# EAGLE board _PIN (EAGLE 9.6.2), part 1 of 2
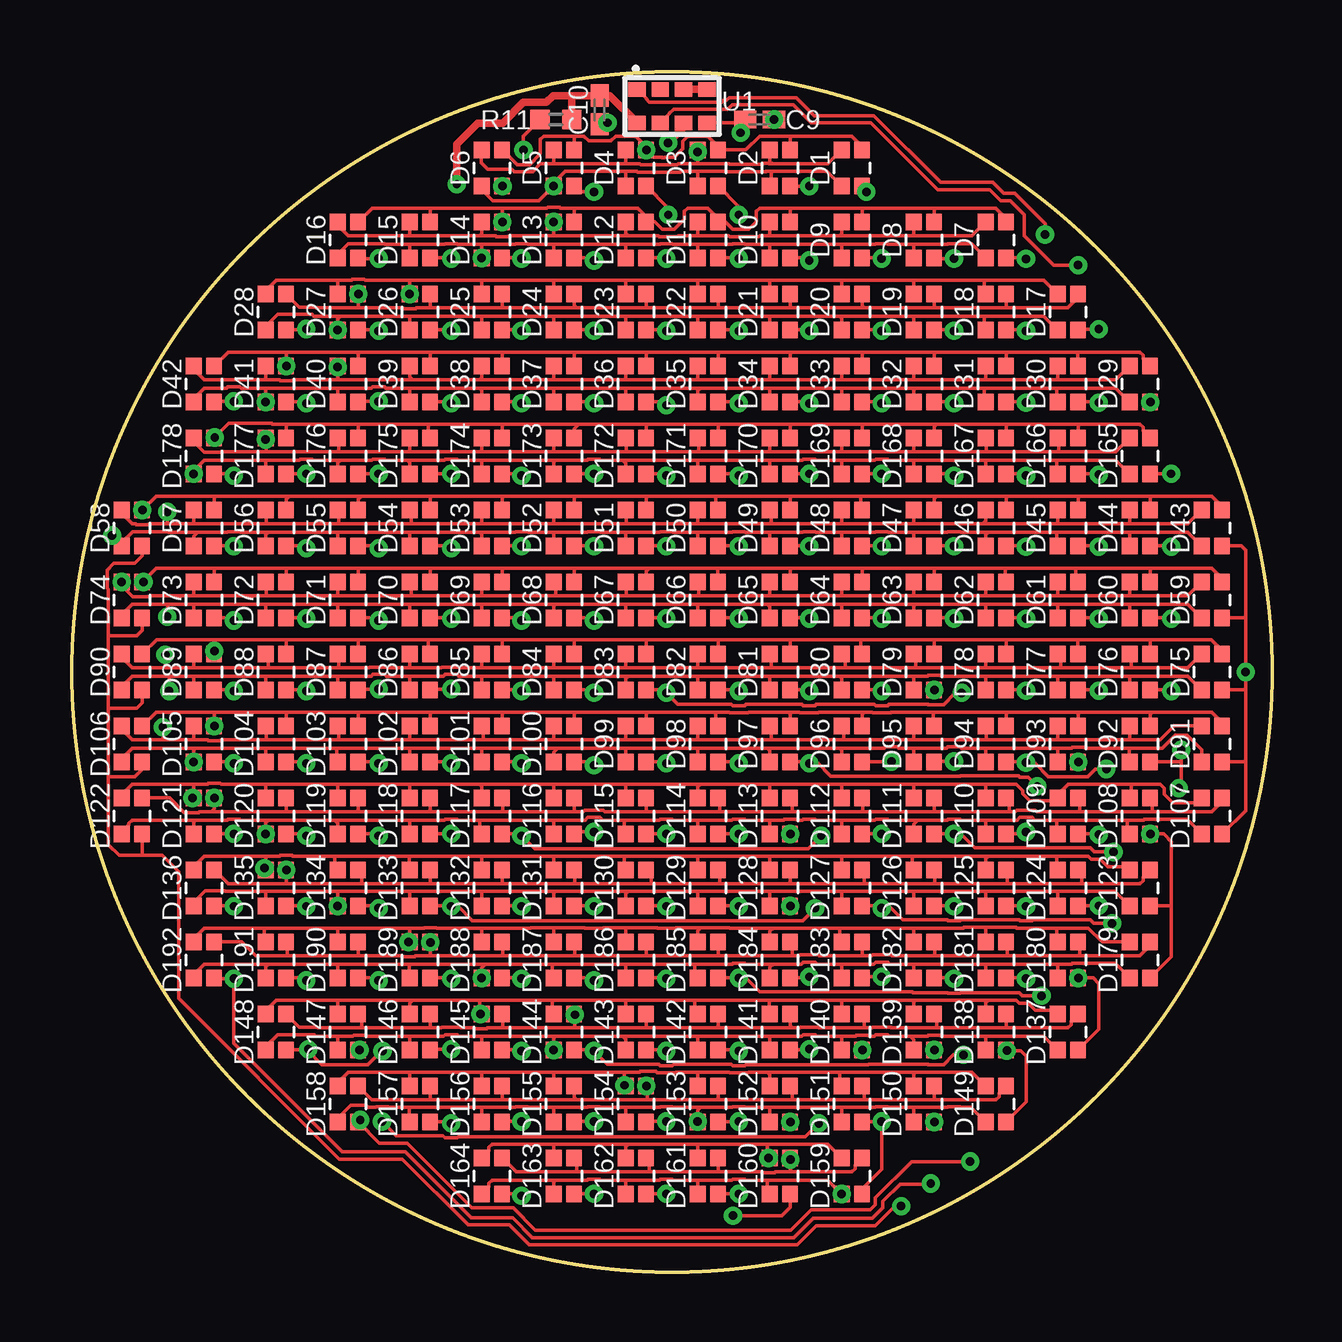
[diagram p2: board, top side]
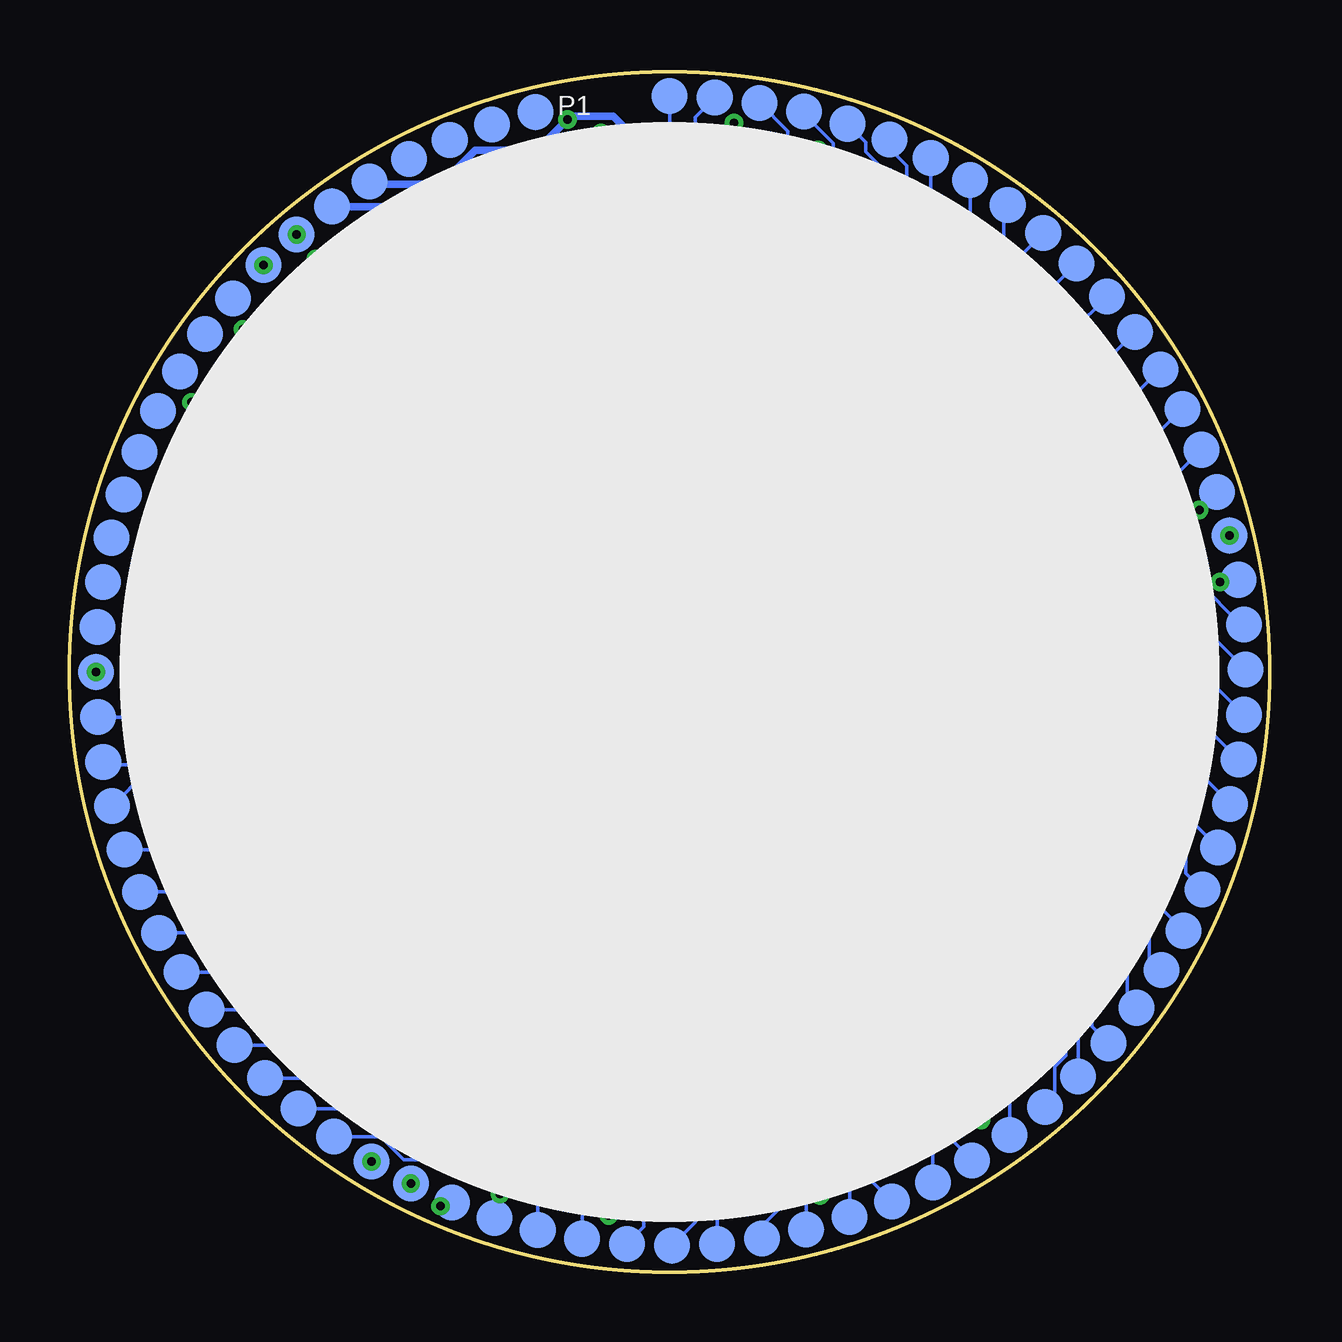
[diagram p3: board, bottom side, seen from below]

Size 50 x 50 mm. Coordinates in mm from the lower left corner, seen from the top.
Outline: circle at 25,25 radius 25
Copper layers (1*16): Top 0.035mm / dielectric 0.8mm / Bottom 0.035mm
Design rules "default *": minimum track width 6mil, minimum drill 0.35mm, track to track 6mil, track to pad 6mil, pad to pad 6mil, via to via 6mil, smd to smd 6mil, copper to edge 6mil, drill to drill 6mil, minimum pad ring 10mil, minimum via ring 8mil, stop-mask expansion 4mil, vias tented up to drill 0.35mm, thermal gap 6mil

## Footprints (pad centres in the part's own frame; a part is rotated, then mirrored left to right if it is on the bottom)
C0402K = smd 0.925 x 0.74: 1 -0.6,0; 2 0.6,0
LED_RGB_0603 = smd 0.65 x 0.7: 1 -0.425,-0.75; 2 0.425,-0.75; 3 0.425,0.75; 4 -0.425,0.75
CONNECTOR_61 = smd 1.5 x 1.5: 1 -24,0; 2 -23.93,1.879; 3 -23.713,3.747; 4 -23.35,5.593; 5 -22.843,7.404; 6 -22.195,9.17; 7 -21.412,10.879; 8 -20.496,12.522; 9 -19.454,14.088; 10 -18.293,15.567; 11 -17.019,16.95; 12 -15.641,18.23; 13 -14.166,19.397; 14 -12.605,20.445; 15 -10.966,21.367; 16 -9.259,22.158; 17 -7.496,22.813; 18 -5.687,23.327; 19 -3.843,23.698; 20 -1.976,23.922; 21 -0.097,24; 22 1.782,23.93; 23 3.65,23.713; 24 5.495,23.35; 25 7.307,22.843; 26 9.072,22.195; 27 10.782,21.412; 28 12.425,20.496; 29 13.99,19.454; 30 15.47,18.293; 31 16.853,17.019; 32 18.133,15.641; 33 19.3,14.166; 34 20.348,12.605; 35 21.27,10.966; 36 22.061,9.259; 37 22.716,7.496; 38 23.23,5.687; 39 23.6,3.844; 40 23.825,1.976; 41 23.903,0.097; 42 23.833,-1.782; 43 23.616,-3.65; 44 23.252,-5.495; 45 22.746,-7.306; 46 22.098,-9.072; 47 21.314,-10.782; 48 20.399,-12.424; 49 19.357,-13.99; 50 18.196,-15.47; 51 16.922,-16.853; 52 15.544,-18.133; 53 14.069,-19.3; 54 12.507,-20.348; 55 10.868,-21.27; 56 9.162,-22.061; 57 7.399,-22.715; 58 5.59,-23.23; 59 3.746,-23.6; 60 1.879,-23.825; 61 0,-23.903; 62 -1.879,-23.833; 63 -3.747,-23.615; 64 -5.593,-23.252; 65 -7.404,-22.746; 66 -9.169,-22.098; 67 -10.879,-21.314; 68 -12.522,-20.399; 69 -14.088,-19.357; 70 -15.567,-18.196; 71 -16.95,-16.922; 72 -18.23,-15.544; 73 -19.397,-14.069; 74 -20.445,-12.507; 75 -21.367,-10.868; 76 -22.158,-9.162; 77 -22.813,-7.399; 78 -23.327,-5.59
R0402 = smd 0.8 x 0.8: 1 -0.659,0; 2 0.659,0
APDS-9950 = smd 0.6 x 0.72: 1 0.7,1.455; 2 0.7,0.485; 3 0.7,-0.485; 4 0.7,-1.455; 5 -0.7,-1.455; 6 -0.7,-0.485; 7 -0.7,0.485; 8 -0.7,1.455

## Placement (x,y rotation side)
C9  100n  [C0402K]  28.65,48.02 180 top
C10  100n  [C0402K]  21.99,48.42 90 top
D1  LED_RGB_0603  [LED_RGB_0603]  32.5,46 0 top
D2  LED_RGB_0603  [LED_RGB_0603]  29.5,46 0 top
D3  LED_RGB_0603  [LED_RGB_0603]  26.5,46 0 top
D4  LED_RGB_0603  [LED_RGB_0603]  23.5,46 0 top
D5  LED_RGB_0603  [LED_RGB_0603]  20.5,46 0 top
D6  LED_RGB_0603  [LED_RGB_0603]  17.5,46 0 top
D7  LED_RGB_0603  [LED_RGB_0603]  38.5,43 0 top
D8  LED_RGB_0603  [LED_RGB_0603]  35.5,43 0 top
D9  LED_RGB_0603  [LED_RGB_0603]  32.5,43 0 top
D10  LED_RGB_0603  [LED_RGB_0603]  29.5,43 0 top
D11  LED_RGB_0603  [LED_RGB_0603]  26.5,43 0 top
D12  LED_RGB_0603  [LED_RGB_0603]  23.5,43 0 top
D13  LED_RGB_0603  [LED_RGB_0603]  20.5,43 0 top
D14  LED_RGB_0603  [LED_RGB_0603]  17.5,43 0 top
D15  LED_RGB_0603  [LED_RGB_0603]  14.5,43 0 top
D16  LED_RGB_0603  [LED_RGB_0603]  11.5,43 0 top
D17  LED_RGB_0603  [LED_RGB_0603]  41.5,40 0 top
D18  LED_RGB_0603  [LED_RGB_0603]  38.5,40 0 top
D19  LED_RGB_0603  [LED_RGB_0603]  35.5,40 0 top
D20  LED_RGB_0603  [LED_RGB_0603]  32.5,40 0 top
D21  LED_RGB_0603  [LED_RGB_0603]  29.5,40 0 top
D22  LED_RGB_0603  [LED_RGB_0603]  26.5,40 0 top
D23  LED_RGB_0603  [LED_RGB_0603]  23.5,40 0 top
D24  LED_RGB_0603  [LED_RGB_0603]  20.5,40 0 top
D25  LED_RGB_0603  [LED_RGB_0603]  17.5,40 0 top
D26  LED_RGB_0603  [LED_RGB_0603]  14.5,40 0 top
D27  LED_RGB_0603  [LED_RGB_0603]  11.5,40 0 top
D28  LED_RGB_0603  [LED_RGB_0603]  8.5,40 0 top
D29  LED_RGB_0603  [LED_RGB_0603]  44.5,37 0 top
D30  LED_RGB_0603  [LED_RGB_0603]  41.5,37 0 top
D31  LED_RGB_0603  [LED_RGB_0603]  38.5,37 0 top
D32  LED_RGB_0603  [LED_RGB_0603]  35.5,37 0 top
D33  LED_RGB_0603  [LED_RGB_0603]  32.5,37 0 top
D34  LED_RGB_0603  [LED_RGB_0603]  29.5,37 0 top
D35  LED_RGB_0603  [LED_RGB_0603]  26.5,37 0 top
D36  LED_RGB_0603  [LED_RGB_0603]  23.5,37 0 top
D37  LED_RGB_0603  [LED_RGB_0603]  20.5,37 0 top
D38  LED_RGB_0603  [LED_RGB_0603]  17.5,37 0 top
D39  LED_RGB_0603  [LED_RGB_0603]  14.5,37 0 top
D40  LED_RGB_0603  [LED_RGB_0603]  11.5,37 0 top
D41  LED_RGB_0603  [LED_RGB_0603]  8.5,37 0 top
D42  LED_RGB_0603  [LED_RGB_0603]  5.5,37 0 top
D43  LED_RGB_0603  [LED_RGB_0603]  47.5,31 0 top
D44  LED_RGB_0603  [LED_RGB_0603]  44.5,31 0 top
D45  LED_RGB_0603  [LED_RGB_0603]  41.5,31 0 top
D46  LED_RGB_0603  [LED_RGB_0603]  38.5,31 0 top
D47  LED_RGB_0603  [LED_RGB_0603]  35.5,31 0 top
D48  LED_RGB_0603  [LED_RGB_0603]  32.5,31 0 top
D49  LED_RGB_0603  [LED_RGB_0603]  29.5,31 0 top
D50  LED_RGB_0603  [LED_RGB_0603]  26.5,31 0 top
D51  LED_RGB_0603  [LED_RGB_0603]  23.5,31 0 top
D52  LED_RGB_0603  [LED_RGB_0603]  20.5,31 0 top
D53  LED_RGB_0603  [LED_RGB_0603]  17.5,31 0 top
D54  LED_RGB_0603  [LED_RGB_0603]  14.5,31 0 top
D55  LED_RGB_0603  [LED_RGB_0603]  11.5,31 0 top
D56  LED_RGB_0603  [LED_RGB_0603]  8.5,31 0 top
D57  LED_RGB_0603  [LED_RGB_0603]  5.5,31 0 top
D58  LED_RGB_0603  [LED_RGB_0603]  2.5,31 0 top
D59  LED_RGB_0603  [LED_RGB_0603]  47.5,28 0 top
D60  LED_RGB_0603  [LED_RGB_0603]  44.5,28 0 top
D61  LED_RGB_0603  [LED_RGB_0603]  41.5,28 0 top
D62  LED_RGB_0603  [LED_RGB_0603]  38.5,28 0 top
D63  LED_RGB_0603  [LED_RGB_0603]  35.5,28 0 top
D64  LED_RGB_0603  [LED_RGB_0603]  32.5,28 0 top
D65  LED_RGB_0603  [LED_RGB_0603]  29.5,28 0 top
D66  LED_RGB_0603  [LED_RGB_0603]  26.5,28 0 top
D67  LED_RGB_0603  [LED_RGB_0603]  23.5,28 0 top
D68  LED_RGB_0603  [LED_RGB_0603]  20.5,28 0 top
D69  LED_RGB_0603  [LED_RGB_0603]  17.5,28 0 top
D70  LED_RGB_0603  [LED_RGB_0603]  14.5,28 0 top
D71  LED_RGB_0603  [LED_RGB_0603]  11.5,28 0 top
D72  LED_RGB_0603  [LED_RGB_0603]  8.5,28 0 top
D73  LED_RGB_0603  [LED_RGB_0603]  5.5,28 0 top
D74  LED_RGB_0603  [LED_RGB_0603]  2.5,28 0 top
D75  LED_RGB_0603  [LED_RGB_0603]  47.5,25 0 top
D76  LED_RGB_0603  [LED_RGB_0603]  44.5,25 0 top
D77  LED_RGB_0603  [LED_RGB_0603]  41.5,25 0 top
D78  LED_RGB_0603  [LED_RGB_0603]  38.5,25 0 top
D79  LED_RGB_0603  [LED_RGB_0603]  35.5,25 0 top
D80  LED_RGB_0603  [LED_RGB_0603]  32.5,25 0 top
D81  LED_RGB_0603  [LED_RGB_0603]  29.5,25 0 top
D82  LED_RGB_0603  [LED_RGB_0603]  26.5,25 0 top
D83  LED_RGB_0603  [LED_RGB_0603]  23.5,25 0 top
D84  LED_RGB_0603  [LED_RGB_0603]  20.5,25 0 top
D85  LED_RGB_0603  [LED_RGB_0603]  17.5,25 0 top
D86  LED_RGB_0603  [LED_RGB_0603]  14.5,25 0 top
D87  LED_RGB_0603  [LED_RGB_0603]  11.5,25 0 top
D88  LED_RGB_0603  [LED_RGB_0603]  8.5,25 0 top
D89  LED_RGB_0603  [LED_RGB_0603]  5.5,25 0 top
D90  LED_RGB_0603  [LED_RGB_0603]  2.5,25 0 top
D91  LED_RGB_0603  [LED_RGB_0603]  47.5,22 0 top
D92  LED_RGB_0603  [LED_RGB_0603]  44.5,22 0 top
D93  LED_RGB_0603  [LED_RGB_0603]  41.5,22 0 top
D94  LED_RGB_0603  [LED_RGB_0603]  38.5,22 0 top
D95  LED_RGB_0603  [LED_RGB_0603]  35.5,22 0 top
D96  LED_RGB_0603  [LED_RGB_0603]  32.5,22 0 top
D97  LED_RGB_0603  [LED_RGB_0603]  29.5,22 0 top
D98  LED_RGB_0603  [LED_RGB_0603]  26.5,22 0 top
D99  LED_RGB_0603  [LED_RGB_0603]  23.5,22 0 top
D100  LED_RGB_0603  [LED_RGB_0603]  20.5,22 0 top
D101  LED_RGB_0603  [LED_RGB_0603]  17.5,22 0 top
D102  LED_RGB_0603  [LED_RGB_0603]  14.5,22 0 top
D103  LED_RGB_0603  [LED_RGB_0603]  11.5,22 0 top
D104  LED_RGB_0603  [LED_RGB_0603]  8.5,22 0 top
D105  LED_RGB_0603  [LED_RGB_0603]  5.5,22 0 top
D106  LED_RGB_0603  [LED_RGB_0603]  2.5,22 0 top
D107  LED_RGB_0603  [LED_RGB_0603]  47.5,19 0 top
D108  LED_RGB_0603  [LED_RGB_0603]  44.5,19 0 top
D109  LED_RGB_0603  [LED_RGB_0603]  41.5,19 0 top
D110  LED_RGB_0603  [LED_RGB_0603]  38.5,19 0 top
D111  LED_RGB_0603  [LED_RGB_0603]  35.5,19 0 top
D112  LED_RGB_0603  [LED_RGB_0603]  32.5,19 0 top
D113  LED_RGB_0603  [LED_RGB_0603]  29.5,19 0 top
D114  LED_RGB_0603  [LED_RGB_0603]  26.5,19 0 top
D115  LED_RGB_0603  [LED_RGB_0603]  23.5,19 0 top
D116  LED_RGB_0603  [LED_RGB_0603]  20.5,19 0 top
D117  LED_RGB_0603  [LED_RGB_0603]  17.5,19 0 top
D118  LED_RGB_0603  [LED_RGB_0603]  14.5,19 0 top
D119  LED_RGB_0603  [LED_RGB_0603]  11.5,19 0 top
D120  LED_RGB_0603  [LED_RGB_0603]  8.5,19 0 top
D121  LED_RGB_0603  [LED_RGB_0603]  5.5,19 0 top
D122  LED_RGB_0603  [LED_RGB_0603]  2.5,19 0 top
D123  LED_RGB_0603  [LED_RGB_0603]  44.5,16 0 top
D124  LED_RGB_0603  [LED_RGB_0603]  41.5,16 0 top
D125  LED_RGB_0603  [LED_RGB_0603]  38.5,16 0 top
D126  LED_RGB_0603  [LED_RGB_0603]  35.5,16 0 top
D127  LED_RGB_0603  [LED_RGB_0603]  32.5,16 0 top
D128  LED_RGB_0603  [LED_RGB_0603]  29.5,16 0 top
D129  LED_RGB_0603  [LED_RGB_0603]  26.5,16 0 top
D130  LED_RGB_0603  [LED_RGB_0603]  23.5,16 0 top
D131  LED_RGB_0603  [LED_RGB_0603]  20.5,16 0 top
D132  LED_RGB_0603  [LED_RGB_0603]  17.5,16 0 top
D133  LED_RGB_0603  [LED_RGB_0603]  14.5,16 0 top
D134  LED_RGB_0603  [LED_RGB_0603]  11.5,16 0 top
D135  LED_RGB_0603  [LED_RGB_0603]  8.5,16 0 top
D136  LED_RGB_0603  [LED_RGB_0603]  5.5,16 0 top
D137  LED_RGB_0603  [LED_RGB_0603]  41.5,10 0 top
D138  LED_RGB_0603  [LED_RGB_0603]  38.5,10 0 top
D139  LED_RGB_0603  [LED_RGB_0603]  35.5,10 0 top
D140  LED_RGB_0603  [LED_RGB_0603]  32.5,10 0 top
D141  LED_RGB_0603  [LED_RGB_0603]  29.5,10 0 top
D142  LED_RGB_0603  [LED_RGB_0603]  26.5,10 0 top
D143  LED_RGB_0603  [LED_RGB_0603]  23.5,10 0 top
D144  LED_RGB_0603  [LED_RGB_0603]  20.5,10 0 top
D145  LED_RGB_0603  [LED_RGB_0603]  17.5,10 0 top
D146  LED_RGB_0603  [LED_RGB_0603]  14.5,10 0 top
D147  LED_RGB_0603  [LED_RGB_0603]  11.5,10 0 top
D148  LED_RGB_0603  [LED_RGB_0603]  8.5,10 0 top
D149  LED_RGB_0603  [LED_RGB_0603]  38.5,7 0 top
D150  LED_RGB_0603  [LED_RGB_0603]  35.5,7 0 top
D151  LED_RGB_0603  [LED_RGB_0603]  32.5,7 0 top
D152  LED_RGB_0603  [LED_RGB_0603]  29.5,7 0 top
D153  LED_RGB_0603  [LED_RGB_0603]  26.5,7 0 top
D154  LED_RGB_0603  [LED_RGB_0603]  23.5,7 0 top
D155  LED_RGB_0603  [LED_RGB_0603]  20.5,7 0 top
D156  LED_RGB_0603  [LED_RGB_0603]  17.5,7 0 top
D157  LED_RGB_0603  [LED_RGB_0603]  14.5,7 0 top
D158  LED_RGB_0603  [LED_RGB_0603]  11.5,7 0 top
D159  LED_RGB_0603  [LED_RGB_0603]  32.5,4 0 top
D160  LED_RGB_0603  [LED_RGB_0603]  29.5,4 0 top
D161  LED_RGB_0603  [LED_RGB_0603]  26.5,4 0 top
D162  LED_RGB_0603  [LED_RGB_0603]  23.5,4 0 top
D163  LED_RGB_0603  [LED_RGB_0603]  20.5,4 0 top
D164  LED_RGB_0603  [LED_RGB_0603]  17.5,4 0 top
D165  LED_RGB_0603  [LED_RGB_0603]  44.5,34 0 top
D166  LED_RGB_0603  [LED_RGB_0603]  41.5,34 0 top
D167  LED_RGB_0603  [LED_RGB_0603]  38.5,34 0 top
D168  LED_RGB_0603  [LED_RGB_0603]  35.5,34 0 top
D169  LED_RGB_0603  [LED_RGB_0603]  32.5,34 0 top
D170  LED_RGB_0603  [LED_RGB_0603]  29.5,34 0 top
D171  LED_RGB_0603  [LED_RGB_0603]  26.5,34 0 top
D172  LED_RGB_0603  [LED_RGB_0603]  23.5,34 0 top
D173  LED_RGB_0603  [LED_RGB_0603]  20.5,34 0 top
D174  LED_RGB_0603  [LED_RGB_0603]  17.5,34 0 top
D175  LED_RGB_0603  [LED_RGB_0603]  14.5,34 0 top
D176  LED_RGB_0603  [LED_RGB_0603]  11.5,34 0 top
D177  LED_RGB_0603  [LED_RGB_0603]  8.5,34 0 top
D178  LED_RGB_0603  [LED_RGB_0603]  5.5,34 0 top
D179  LED_RGB_0603  [LED_RGB_0603]  44.5,13 0 top
D180  LED_RGB_0603  [LED_RGB_0603]  41.5,13 0 top
D181  LED_RGB_0603  [LED_RGB_0603]  38.5,13 0 top
D182  LED_RGB_0603  [LED_RGB_0603]  35.5,13 0 top
D183  LED_RGB_0603  [LED_RGB_0603]  32.5,13 0 top
D184  LED_RGB_0603  [LED_RGB_0603]  29.5,13 0 top
D185  LED_RGB_0603  [LED_RGB_0603]  26.5,13 0 top
D186  LED_RGB_0603  [LED_RGB_0603]  23.5,13 0 top
D187  LED_RGB_0603  [LED_RGB_0603]  20.5,13 0 top
D188  LED_RGB_0603  [LED_RGB_0603]  17.5,13 0 top
D189  LED_RGB_0603  [LED_RGB_0603]  14.5,13 0 top
D190  LED_RGB_0603  [LED_RGB_0603]  11.5,13 0 top
D191  LED_RGB_0603  [LED_RGB_0603]  8.5,13 0 top
D192  LED_RGB_0603  [LED_RGB_0603]  5.5,13 0 top
P1  CON_ROUND  [CONNECTOR_61]  25,25 270 bottom
R11  DNP  [R0402]  20.16,48.02 0 top
U1  APDS-9960  [APDS-9950]  25,48.58 90 top

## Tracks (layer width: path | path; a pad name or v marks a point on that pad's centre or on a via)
+3V3  (via drill 0.35)
  Top 0.305: U1.8 22.4,49.02 C10.2 20.8,49.02 | v16.03,45.32 16.03,46.99 16.91,47.86 17.94,47.86 18.81,48.74 19.76,48.74 20.05,49.02 20.8,49.02 | R11.2 20.82,48.99 20.8,49.02
  Bottom 0.305: P1.73 34.79,44.39 32.91,46.28 29.29,46.28 28.23,45.21 22.51,45.21 22.03,45.69 21.47,45.69 21.07,45.29 21.07,43.61 20.52,43.07 19.56,43.07 19.21,43.42 19.21,43.97 18.62,44.55 18.62,45.53 18.22,45.93 16.64,45.93 v16.03,45.32
B0  (via drill 0.35)
  Top 0.152: D2.3 29.93,47.33 | D1.3 32.92,46.9 32.49,47.33 29.93,47.33 | D4.3 | D4.3 23.93,46.89 23.5,47.33 22.65,47.33 22.45,47.13 21.52,47.13 21.32,47.33 20.93,47.33 | D4.3 24.24,46.44 24.6,46.44 24.6,46.43 24.69,46.43 24.69,46.44 25.09,46.44 25.45,46.8 25.45,47.12 25.66,47.33 26.5,47.33 26.93,46.9 D3.3 28.08,46.75 28.66,47.33 29.93,47.33 | D6.3 17.96,46.75 18.56,46.15 19.06,46.15 19.52,46.6 19.52,47.2 19.66,47.33 20.93,47.33 | D5.3 20.93,47.33
  Bottom 0.152: P1.2 23.93,48.12 D4.3
  other vias: 23.93,46.75
B1  (via drill 0.35)
  Top 0.152: D16.3 12.5,44.33 14.92,44.33 | D7.3 38.92,43.9 38.49,44.33 35.96,44.33 | 20.95,44.33 23.57,44.33 23.93,43.98 D12.3 24.29,43.75 24.59,43.45 25.1,43.45 25.52,43.87 25.52,44.2 25.66,44.33 26.5,44.33 26.93,43.9 D11.3 27.23,43.75 27.53,43.45 28.21,43.45 28.52,43.76 28.52,44.2 28.66,44.33 29.92,44.33 | 29.92,44.33 32.94,44.33 | 32.94,44.33 35.96,44.33 | D8.3 35.92,44.3 35.96,44.33 | D9.3 32.92,44.31 32.94,44.33 | D10.3 29.93,44.33 29.92,44.33 | D13.3 20.93,44.3 20.95,44.33 | D15.3 14.93,44.33 14.92,44.33 | 20.95,44.33 20.35,44.33 20.32,44.36 19.82,44.36 19.79,44.33 17.94,44.33 | D14.3 17.93,44.31 17.94,44.33 | 14.92,44.33 17.94,44.33
  Bottom 0.152: P1.5 16.83,47.07 16.83,46.67 16.09,45.93 15.78,45.93 15.43,45.57 15.43,44.99 16.67,43.75 D14.3
  other vias: 17.93,43.75
B2  (via drill 0.35)
  Top 0.152: D17.3 41.92,40.6 41.49,40.17 38.97,40.17 | 14.92,40.17 17.86,40.17 | 17.86,40.17 21.03,40.17 | 21.03,40.17 23.89,40.17 | 23.89,40.17 26.91,40.17 | 26.91,40.17 29.92,40.17 | 29.92,40.17 33.02,40.17 | 33.02,40.17 35.96,40.17 | 35.96,40.17 38.97,40.17 | D18.3 38.92,40.22 38.97,40.17 | D19.3 35.92,40.2 35.96,40.17 | D20.3 32.92,40.27 33.02,40.17 | D21.3 29.93,40.17 29.92,40.17 | D22.3 26.93,40.19 26.91,40.17 | D23.3 23.93,40.2 23.89,40.17 | D24.3 20.93,40.28 21.03,40.17 | D25.3 17.93,40.24 17.86,40.17 | D26.3 14.93,40.17 14.92,40.17 | D27.3 | 11.99,40.17 11.93,40.23 D27.3 | D28.3 9.47,40.2 10.14,40.2 10.17,40.17 11.99,40.17 | 11.99,40.17 13.79,40.17 13.82,40.14 14.32,40.14 14.35,40.17 14.92,40.17 | D27.3
  Bottom 0.152: P1.8 12.48,43.58 11.93,43.03 D27.3
  other vias: 11.93,40.75
B3  (via drill 0.35)
  Top 0.152: D42.3 6.5,38.33 8.97,38.33 | D29.3 44.63,38.05 44.63,38.2 44.49,38.33 41.91,38.33 | 8.97,38.33 11.83,38.33 | 11.83,38.33 14.92,38.33 | 14.92,38.33 17.94,38.33 | 17.94,38.33 20.88,38.33 | 20.88,38.33 23.89,38.33 | 23.89,38.33 26.99,38.33 | 26.99,38.33 29.92,38.33 | 29.92,38.33 32.94,38.33 | 32.94,38.33 35.96,38.33 | 35.96,38.33 38.97,38.33 | 38.97,38.33 41.91,38.33 | D30.3 41.91,37.77 41.91,38.33 | D31.3 38.92,38.28 38.97,38.33 | D32.3 35.92,38.3 35.96,38.33 | D33.3 32.92,38.31 32.94,38.33 | D34.3 29.93,38.33 29.92,38.33 | D35.3 26.93,38.27 26.99,38.33 | D36.3 23.93,38.3 23.89,38.33 | D37.3 20.93,38.28 20.88,38.33 | D38.3 17.93,38.31 17.94,38.33 | D39.3 14.93,38.33 14.92,38.33 | D40.3 11.93,38.23 11.83,38.33 | D41.3 | 8.97,38.33 8.93,38.28 8.93,37.94 D41.3 | D41.3
  Bottom 0.152: P1.11 8.93,41.14 D41.3
  other vias: 8.93,37.75
B4  (via drill 0.35)
  Top 0.152: D165.3 44.63,35.05 44.63,35.2 44.49,35.33 41.91,35.33 | 41.91,35.33 38.97,35.33 | 38.97,35.33 36.04,35.33 | 36.04,35.33 32.94,35.33 | 32.94,35.33 30,35.33 | 30,35.33 26.91,35.33 | 26.91,35.33 23.89,35.33 | 23.89,35.33 21.11,35.33 | 21.11,35.33 17.94,35.33 | 17.94,35.33 14.84,35.33 | 14.84,35.33 11.99,35.33 | 11.99,35.33 8.89,35.33 | D166.3 41.92,35.31 41.91,35.33 | D167.3 38.92,35.28 38.97,35.33 | D168.3 35.92,35.22 36.04,35.33 | D169.3 32.92,35.31 32.94,35.33 | D170.3 29.93,35.25 30,35.33 | D171.3 26.93,35.31 26.91,35.33 | D172.3 23.93,35.3 23.89,35.33 | D174.3 17.93,35.31 17.94,35.33 | D175.3 14.84,34.83 14.84,35.33 | D176.3 11.93,35.27 11.99,35.33 | D177.3 8.93,35.29 8.89,35.33 | D173.3 20.93,35.14 21.11,35.33 | 8.89,35.33 8.35,35.33 8.32,35.36 6.53,35.36 v5.95,34.77 D178.3
  Bottom 0.152: P1.14 5.95,36.21 v5.95,34.77
B5  (via drill 0.35)
  Top 0.152: D43.3 47.92,31.9 47.49,32.33 44.93,32.33 | 5.95,32.33 9.05,32.33 | 9.05,32.33 12.06,32.33 | 12.06,32.33 15,32.33 | 15,32.33 17.94,32.33 | 17.94,32.33 20.95,32.33 | 20.95,32.33 23.89,32.33 | 23.89,32.33 26.83,32.33 | 26.83,32.33 30,32.33 | 30,32.33 32.86,32.33 | 32.86,32.33 36.04,32.33 | 36.04,32.33 38.89,32.33 | 38.89,32.33 41.99,32.33 | 41.99,32.33 44.93,32.33 | D55.3 11.93,32.19 12.06,32.33 | D54.3 14.93,32.25 15,32.33 | D53.3 17.93,32.31 17.94,32.33 | D52.3 20.93,32.3 20.95,32.33 | D51.3 23.93,32.3 23.89,32.33 | D50.3 26.83,31.85 26.83,32.33 | D48.3 32.86,31.81 32.86,32.33 | D47.3 35.92,32.22 36.04,32.33 | D46.3 38.92,32.3 38.89,32.33 | D45.3 41.92,32.26 41.99,32.33 | D44.3 44.92,32.33 44.93,32.33 | D49.3 29.93,32.25 30,32.33 | D57.3 5.92,32.3 5.95,32.33 | D56.3 8.93,32.2 9.05,32.33 | D58.3 v2.93,31.76 | v2.93,31.75 v2.93,31.76 | 5.95,32.33 3.5,32.33 v2.93,31.76
  Bottom 0.152: P1.17 v2.93,31.75
B6  (via drill 0.35)
  Top 0.152: D59.3 47.92,28.9 47.49,29.33 44.93,29.33 | 2.98,28.8 3.5,29.33 5.95,29.33 | 2.98,28.8 D74.3 | 44.93,29.33 41.83,29.33 | 41.83,29.33 38.89,29.33 | 38.89,29.33 35.96,29.33 | 35.96,29.33 32.94,29.33 | 32.94,29.33 29.92,29.33 | 29.92,29.33 26.91,29.33 | 26.91,29.33 24.05,29.33 | 24.05,29.33 20.88,29.33 | 20.88,29.33 17.94,29.33 | 17.94,29.33 15,29.33 | 15,29.33 11.99,29.33 | 11.99,29.33 8.97,29.33 | 8.97,29.33 5.95,29.33 | D73.3 5.92,29.3 5.95,29.33 | D72.3 8.93,29.28 8.97,29.33 | D71.3 11.93,29.27 11.99,29.33 | D70.3 14.93,29.25 15,29.33 | D69.3 17.93,29.32 17.94,29.33 | D68.3 20.93,29.28 20.88,29.33 | D67.3 23.93,29.2 24.05,29.33 | D60.3 44.92,29.33 44.93,29.33 | D61.3 41.83,28.84 41.83,29.33 | D62.3 38.89,28.78 38.89,29.33 | D63.3 35.92,29.3 35.96,29.33 | D64.3 32.92,29.31 32.94,29.33 | D65.3 29.92,29.33 | D66.3 26.91,28.77 26.91,29.33 | v2.98,28.75 2.98,28.8
  Bottom 0.152: P1.20 1.2,26.98 v2.98,28.75
B7  (via drill 0.35)
  Top 0.152: D90.3 3.53,26.35 5.95,26.35 | D75.3 47.92,25.9 47.47,26.35 44.93,26.35 | 5.95,26.35 8.97,26.35 | 8.97,26.35 11.99,26.35 | 11.99,26.35 14.84,26.35 | 14.84,26.35 17.94,26.35 | 17.94,26.35 20.95,26.35 | 20.95,26.35 23.97,26.35 | 23.97,26.35 26.91,26.35 | 26.91,26.35 29.92,26.35 | 29.92,26.35 32.86,26.35 | 32.86,26.35 35.96,26.35 | 35.96,26.35 38.97,26.35 | 38.97,26.35 41.91,26.35 | 41.91,26.35 44.93,26.35 | 5.95,26.35 5.92,26.32 D89.3 v5.92,25.87 v5.93,25.88 | D88.3 8.93,26.31 8.97,26.35 | D87.3 11.93,26.29 11.99,26.35 | D86.3 14.84,25.83 14.84,26.35 | D85.3 17.93,26.34 17.94,26.35 | D84.3 20.93,26.32 20.95,26.35 | D77.3 41.91,25.77 41.91,26.35 | D76.3 44.92,26.35 44.93,26.35 | D78.3 38.92,26.3 38.97,26.35 | D79.3 35.92,26.32 35.96,26.35 | D80.3 32.86,25.81 32.86,26.35 | D81.3 29.92,26.35 | D83.3 23.93,26.31 23.97,26.35 | D82.3 26.93,26.34 26.91,26.35
  Bottom 0.152: v5.93,25.88 5.81,25.88 4.75,24.82 3.8,24.82 2.55,23.57 2.55,22.61 P1.23
B8  (via drill 0.35)
  Top 0.152: D106.3 3.5,23.33 5.95,23.33 | D91.3 47.92,22.9 47.49,23.33 45.01,23.33 | 5.95,23.33 8.97,23.33 | 8.97,23.33 11.99,23.33 | 11.99,23.33 14.92,23.33 | 14.92,23.33 17.94,23.33 | 17.94,23.33 20.95,23.33 | 20.95,23.33 23.89,23.33 | 23.89,23.33 26.83,23.33 | 35.88,23.33 38.97,23.33 | 38.97,23.33 41.83,23.33 | 41.83,23.33 45.01,23.33 | D105.3 | D105.3 5.92,23.3 5.95,23.33 | D104.3 8.93,23.28 8.97,23.33 | D103.3 11.93,23.27 11.99,23.33 | D102.3 14.92,23.33 | D101.3 17.93,23.32 17.94,23.33 | D100.3 20.93,23.3 20.95,23.33 | D99.3 23.93,23.3 23.89,23.33 | D98.3 26.83,22.85 26.83,23.33 | D96.3 32.92,23.23 33.02,23.33 | D97.3 29.93,23.25 29.84,23.33 | D95.3 35.88,22.8 35.88,23.33 | D94.3 38.92,23.28 38.97,23.33 | D93.3 41.92,23.23 41.83,23.33 | D92.3 44.92,23.25 45.01,23.33 | 33.02,23.33 33.33,23.33 33.36,23.3 34.11,23.3 34.14,23.33 35.88,23.33 | 29.84,23.33 30.31,23.33 30.34,23.3 31.1,23.3 31.13,23.33 33.02,23.33 | 26.83,23.33 27.37,23.33 27.4,23.3 28.16,23.3 28.19,23.33 29.84,23.33 | v5.93,22.75 D105.3
  Bottom 0.152: P1.26 3.49,16.62 3.49,21.55 4.39,22.45 4.39,22.46 4.67,22.75 v5.93,22.75
B9  (via drill 0.35)
  Top 0.152: D122.3 4.08,19.75 4.68,19.14 5.27,19.14 5.3,19.17 5.79,19.17 | D107.3 47.92,19.6 47.49,19.17 45.01,19.17 | 5.79,19.17 8.89,19.17 | 8.89,19.17 11.83,19.17 | 11.83,19.17 14.84,19.17 | 14.84,19.17 17.94,19.17 | 17.94,19.17 20.88,19.17 | 23.89,19.17 26.99,19.17 | 26.99,19.17 30,19.17 | 30,19.17 32.94,19.17 | 32.94,19.17 35.96,19.17 | 35.96,19.17 39.05,19.17 | 41.99,19.17 45.01,19.17 | D120.3 8.93,19.21 8.89,19.17 | 5.79,19.17 5.92,19.3 D121.3 v5.93,19.75 | D119.3 11.93,19.27 11.83,19.17 | D118.3 14.93,19.25 14.84,19.17 | D117.3 17.94,19.74 17.94,19.17 | D116.3 20.93,19.22 20.88,19.17 | D115.3 23.93,19.2 23.89,19.17 | D114.3 26.99,19.69 26.99,19.17 | D113.3 30,19.67 30,19.17 | D112.3 32.94,19.73 32.94,19.17 | D111.3 35.92,19.2 35.96,19.17 | D110.3 39.05,19.62 39.05,19.17 | D109.3 41.99,19.69 41.99,19.17 | D108.3 45.01,19.67 45.01,19.17 | 39.05,19.17 39.3,19.17 39.37,19.25 40.13,19.25 40.2,19.17 41.99,19.17 | 20.88,19.17 21.3,19.17 21.37,19.25 22.13,19.25 22.2,19.17 23.89,19.17
  Bottom 0.152: v5.93,19.75 5.93,11.39 P1.29
B10  (via drill 0.35)
  Top 0.152: D123.3 44.63,16.45 44.63,16.3 44.49,16.17 42.07,16.17 | D136.3 6.5,16.17 8.89,16.17 | 42.07,16.17 38.97,16.17 | 38.97,16.17 35.96,16.17 | 35.96,16.17 33.02,16.17 | 33.02,16.17 29.84,16.17 | 29.84,16.17 26.99,16.17 | 26.99,16.17 24.13,16.17 | 24.13,16.17 20.95,16.17 | 20.95,16.17 17.94,16.17 | 17.94,16.17 14.92,16.17 | 14.92,16.17 12.06,16.17 | 12.06,16.17 8.89,16.17 | D135.3 | D135.3 8.93,16.21 8.89,16.17 | D134.3 12.06,16.61 12.06,16.17 | D133.3 14.93,16.17 14.92,16.17 | D132.3 17.93,16.18 17.94,16.17 | D131.3 20.95,16.72 20.95,16.17 | D130.3 24.13,16.55 24.13,16.17 | D129.3 26.99,16.69 26.99,16.17 | D128.3 29.93,16.25 29.84,16.17 | D127.3 33.02,16.66 33.02,16.17 | D126.3 35.96,16.72 35.96,16.17 | D125.3 38.97,16.7 38.97,16.17 | D124.3 42.07,16.61 42.07,16.17 | D135.3
  Bottom 0.152: P1.32 8.96,7.27 8.96,8.55 8.49,9.02 8.49,16.31 D135.3
  other vias: 8.93,16.75
B11  (via drill 0.35)
  Top 0.152: D192.3 7.08,13.75 7.66,13.17 8.97,13.17 | D179.3 44.92,13.6 44.49,13.17 41.99,13.17 | 8.97,13.17 11.91,13.17 | 14.92,13.17 17.94,13.17 | 17.94,13.17 20.95,13.17 | 20.95,13.17 23.97,13.17 | 23.97,13.17 26.91,13.17 | 26.91,13.17 30,13.17 | 35.96,13.17 38.97,13.17 | 38.97,13.17 41.99,13.17 | D180.3 41.99,13.69 41.99,13.17 | D181.3 38.97,13.7 38.97,13.17 | D182.3 35.96,13.72 35.96,13.17 | D183.3 32.92,13.23 32.86,13.17 | D184.3 30,13.67 30,13.17 | D185.3 26.93,13.19 26.91,13.17 | D186.3 23.93,13.22 23.97,13.17 | D187.3 20.95,13.72 20.95,13.17 | D188.3 17.94,13.74 17.94,13.17 | D189.3 v14.93,13.73 | v14.93,13.73 14.93,13.17 14.92,13.17 | D190.3 11.93,13.19 11.91,13.17 | D191.3 8.97,13.71 8.97,13.17 | 32.86,13.17 33.31,13.17 33.36,13.21 34.11,13.21 34.16,13.17 35.96,13.17 | 30,13.17 30.3,13.17 30.34,13.21 31.1,13.21 31.14,13.17 32.86,13.17 | v14.93,13.73 | 11.91,13.17 13.74,13.17 13.77,13.14 14.27,13.14 14.3,13.17 14.92,13.17
  Bottom 0.152: P1.35 14.03,12.84 v14.93,13.73
B12  (via drill 0.35)
  Top 0.152: D137.3 41.63,10.45 41.63,10.3 41.49,10.17 38.89,10.17 | 12.06,10.17 14.92,10.17 | 17.94,10.17 20.95,10.17 | 20.95,10.17 23.97,10.17 | 23.97,10.17 26.83,10.17 | 26.83,10.17 30,10.17 | 36.04,10.17 38.89,10.17 | D138.3 38.92,10.2 38.89,10.17 | D139.3 36.04,10.64 36.04,10.17 | D140.3 33.02,10.65 33.02,10.17 | D141.3 29.93,10.25 30,10.17 | D142.3 26.93,10.27 26.83,10.17 | D143.3 23.93,10.22 23.97,10.17 | D144.3 v20.95,10.72 20.95,10.17 | D145.3 | 17.94,10.17 17.94,10.74 D145.3 | D146.3 14.93,10.17 14.92,10.17 | D147.3 12.06,10.61 12.06,10.17 | 33.02,10.17 33.33,10.17 33.36,10.2 34.11,10.2 34.14,10.17 36.04,10.17 | 30,10.17 30.31,10.17 30.34,10.2 31.1,10.2 31.12,10.17 33.02,10.17 | D145.3 | 17.94,10.17 17.3,10.17 17.27,10.14 16.77,10.14 16.74,10.17 16.2,10.17 16.17,10.2 15.42,10.2 15.39,10.17 14.92,10.17 | D148.3 9.48,10.2 10.22,10.2 10.25,10.17 12.06,10.17
  Bottom 0.152: P1.38 19.31,2.9 19.34,2.92 19.34,9.38 20.68,10.72 v20.95,10.72
B13  (via drill 0.35)
  Top 0.152: D149.3 38.63,7.45 38.63,7.3 38.49,7.17 37.14,7.17 37.13,7.18 36.37,7.18 36.36,7.17 35.96,7.17 | 14.92,7.17 17.94,7.17 | 17.94,7.17 18.34,7.17 18.36,7.18 19.11,7.18 19.12,7.17 21.03,7.17 | 30,7.17 33.02,7.17 | 23.97,7.17 23.97,7.46 23.93,7.51 D154.3 | D153.3 26.93,7.27 26.83,7.17 | D157.3 14.93,7.17 14.92,7.17 | 17.93,7.42 D156.3 17.93,7.18 17.94,7.17 | D155.3 20.93,7.28 21.03,7.17 | D154.3 | D152.3 30,7.67 30,7.17 | D151.3 33.02,7.66 33.02,7.17 | D150.3 35.92,7.2 35.96,7.17 | 33.02,7.17 33.35,7.17 33.36,7.18 34.11,7.18 34.12,7.17 35.96,7.17 | 26.83,7.17 27.39,7.17 27.4,7.18 28.16,7.18 28.17,7.17 30,7.17 | D154.3 | 23.97,7.17 24.38,7.17 24.39,7.18 25.14,7.18 25.15,7.17 26.83,7.17 | 21.03,7.17 21.36,7.17 21.37,7.18 22.13,7.18 22.14,7.17 23.97,7.17 | D158.3 12.49,7.18 13.3,7.18 13.31,7.17 14.92,7.17
  Bottom 0.152: P1.41 23.93,2.07 D154.3
  other vias: 23.93,7.75
B14  (via drill 0.35)
  Top 0.152: D164.3 18.5,4.17 21.03,4.17 | D159.3 32.63,4.45 32.63,4.3 32.49,4.17 30,4.17 | 21.03,4.17 24.05,4.17 | 24.05,4.17 26.91,4.17 | D163.3 21.03,4.64 21.03,4.17 | D162.3 24.05,4.62 24.05,4.17 | D161.3 26.93,4.19 26.91,4.17 | 30,4.17 29.93,4.25 D160.3 v29.93,4.68 | 26.91,4.17 28.74,4.17 28.77,4.14 29.27,4.14 29.3,4.17 30,4.17
  Bottom 0.152: P1.44 30.5,4.12 v29.93,4.68
C0  (via drill 0.35)
  Top 0.152: D43.2 48.73,30.25 48.9,30.07 48.9,27.23 | 48.9,27.23 P1.61 48.9,24.21 | 48.9,24.21 48.9,21.27 | 48.9,21.27 48.9,19.23 D107.2 | D91.2 48.88,21.25 48.9,21.27 | D59.2 48.88,27.25 48.9,27.23 | D75.2 48.86,24.25 48.9,24.21
  other vias: 48.9,25
C1  (via drill 0.35)
  Top 0.152: D29.2 v44.93,36.24 | D165.2 44.93,33.26 v45.8,33.26 | D44.2 45.77,30.25 v45.8,30.22 | D60.2 45.77,27.25 v45.8,27.22 | D76.2 45.76,24.25 v45.8,24.21 | D108.2 v44.93,18.25 45.48,18.25 45.8,17.93 45.8,15.24 | 45.8,15.24 45.8,13.12 D179.2 | D123.2 45.79,15.25 45.8,15.24 | D92.2 46.16,21.25 46.22,21.19 | 46.01,20.16 v46.12,20.16 46.22,20.26 46.22,21.19 | v46.22,21.75 46.22,21.19
  Bottom 0.152: v44.93,36.24 44.93,34.13 v45.8,33.26 v45.8,30.22 v45.8,27.22 v45.8,24.21 45.8,23.18 | 45.8,23.18 45.8,22.17 v46.22,21.75 | P1.60 45.86,23.12 45.8,23.18 | v46.12,20.16 44.93,18.98 v44.93,18.25
C2  (via drill 0.35)
  Top 0.152: D17.2 41.96,39.29 v42.78,39.29 | D137.2 42.78,10.11 42.78,12.01 42.55,12.25 v41.93,12.25 D180.2 | D124.2 v42.77,15.25 v42.78,15.26 | D109.2 42.76,18.25 v42.78,18.22 | D77.2 42.76,24.25 v42.78,24.22 | D61.2 42.76,27.25 v42.78,27.22 | D45.2 42.76,30.25 v42.78,30.22 | D166.2 42.76,33.25 v42.78,33.22 | D30.2 42.76,36.25 v42.78,36.22 | D93.2 v41.93,21.25
  Bottom 0.152: v42.78,39.29 v42.78,36.22 v42.78,33.22 v42.78,30.22 v42.78,27.22 v42.78,24.22 41.93,23.37 v41.93,21.25 | v42.78,18.22 42.78,18.18 | 42.78,18.18 42.78,15.32 | 42.78,15.32 v42.78,15.26 | v41.93,21.25 42.54,21.25 42.85,21.56 45.55,21.56 45.97,21.14 48.49,21.14 P1.59 | v41.93,21.25 41.93,19.03 42.78,18.18 | v41.93,12.25 41.93,14.47 42.78,15.32
C3  (via drill 0.35)
  Top 0.152: D7.2 39.71,42.25 v39.75,42.21 | D149.2 39.77,7.09 39.77,8.98 39.53,9.22 v38.95,9.22 D138.2 | D181.2 39.72,12.25 v39.75,12.22 | D125.2 v39.74,15.25 v39.75,15.24 | D94.2 39.72,21.25 v39.75,21.22 40.1,21.22 40.68,20.64 42.32,20.64 42.63,20.95 v43.1,20.95 | D78.2 39.72,24.25 v39.75,24.22 | D62.2 39.72,27.25 v39.75,27.22 | D46.2 39.72,30.25 v39.75,30.22 | D167.2 39.68,33.25 v39.75,33.18 | D31.2 39.72,36.25 v39.75,36.22 | D18.2 39.71,39.25 v39.75,39.21 | D110.2 39.66,18.25 v39.75,18.34
  Bottom 0.152: v39.75,42.21 v39.75,39.21 v39.75,36.22 v39.75,33.18 v39.75,30.22 v39.75,27.22 v39.75,24.22 v39.75,21.22 39.75,20.95 39.61,20.82 39.61,19.75 39.75,19.61 v39.75,18.34 v39.75,15.24 v39.75,12.22 38.95,11.42 v38.95,9.22 | v43.1,20.95 45.72,20.95 45.84,20.84 46.8,20.84 P1.58
C4  (via drill 0.35)
  Top 0.152: v43.4,17.5 42.6,17.5 42.43,17.67 37.62,17.67 37.04,18.25 v36.75,18.25 D111.2 | D182.2 36.72,12.25 v36.75,12.22 | D126.2 v36.74,15.25 v36.75,15.24 | v36.75,42.23 35.95,42.23 D8.2 | D19.2 36.71,39.25 v36.75,39.21 | D32.2 36.7,36.25 v36.75,36.2 | D168.2 36.68,33.25 v36.75,33.18 | D47.2 v36.74,30.25 v36.75,30.24 | D63.2 36.73,27.25 v36.75,27.23 | D95.2 35.95,21.27 v36.75,21.27 | D139.2 v35.93,9.25 | D79.2 v35.93,24.25 | D150.2 v35.93,6.25
  Bottom 0.152: P1.57 43.5,17.6 v43.4,17.5 | v36.75,42.23 v36.75,39.21 v36.75,36.2 v36.75,33.18 v36.75,30.24 v36.75,27.23 35.93,26.41 v35.93,24.25 35.93,22.09 v36.75,21.27 v36.75,18.25 v36.75,15.24 v36.75,12.22 35.93,11.4 v35.93,9.25 35.93,7.78 35.93,7.18 v35.93,6.25
C5  (via drill 0.35)
  Top 0.152: v43.34,14.53 42.58,14.53 42.43,14.67 40.04,14.67 40,14.63 39.5,14.63 39.46,14.67 37.04,14.67 37,14.63 36.5,14.63 36.46,14.67 34.62,14.67 34.04,15.25 D127.2 33.65,15.25 v33.73,15.16 | D151.2 33.71,6.25 v33.73,6.27 33.73,4.27 32.92,3.46 D159.2 | v33.1,45.01 33.1,45.08 D1.2 | D9.2 33.71,42.25 v33.73,42.23 | D20.2 33.7,39.25 v33.73,39.21 | D33.2 33.68,36.25 v33.73,36.2 | D169.2 v33.73,33.25 v33.73,33.26 | D48.2 v33.73,30.25 v33.73,30.24 | D64.2 33.71,27.25 v33.73,27.23 | D80.2 33.69,24.25 v33.73,24.21 | D112.2 v33.73,18.25 v33.73,18.26 | D183.2 32.98,12.3 v33.73,12.3 | D96.2 34.12,21.25 v34.14,21.27 | D140.2 v32.93,9.25
  Bottom 0.152: P1.56 44.65,15.84 v43.34,14.53 | 33.73,21.27 v33.73,18.26 v33.73,15.16 v33.73,12.3 32.93,11.5 v32.93,9.25 32.93,7.07 v33.73,6.27 | 33.73,21.27 v33.73,24.21 v33.73,27.23 v33.73,30.24 v33.73,33.26 v33.73,36.2 v33.73,39.21 v33.73,42.23 33.1,42.86 v33.1,45.01 | v34.14,21.27 33.73,21.27
C6  (via drill 0.35)
  Top 0.152: v40.22,20.24 39.84,20.61 39.5,20.61 39.44,20.67 37.01,20.67 37,20.67 31.62,20.67 31.04,21.25 30.72,21.25 | 30.72,21.25 D97.2 | v30.72,45.24 D2.2 | D10.2 30.62,42.25 v30.72,42.15 | D21.2 30.68,39.25 v30.72,39.21 | D34.2 30.66,36.25 v30.72,36.2 | D170.2 v30.72,33.26 | D49.2 v30.71,30.25 v30.72,30.24 | D65.2 30.69,27.25 v30.72,27.23 | D81.2 30.68,24.25 v30.72,24.21 | 30.72,21.25 v30.72,21.19 | D184.2 30.66,12.25 v30.72,12.3 | D141.2 30.68,9.25 v30.72,9.29 | D113.2 | D160.2 29.93,2.71 29.57,2.35 v27.54,2.35 | D128.2 | D152.2
  Bottom 0.152: P1.55 44.77,14.13 42.28,11.64 41.68,11.64 41.12,12.21 41.12,19.34 v40.22,20.24 | v30.72,45.24 v30.72,42.15 v30.72,39.21 v30.72,36.2 v30.72,33.26 v30.72,30.24 v30.72,27.23 v30.72,24.21 v30.72,21.19 29.93,20.41 D113.2 D128.2 29.93,13.09 v30.72,12.3 v30.72,9.29 30.72,7.04 D152.2 29.66,6.25 28.41,5 28.41,3.03 28.03,2.65 27.84,2.65 v27.54,2.35
  other vias: 29.93,18.25 29.93,15.25 29.93,6.25
C7  (via drill 0.35)
  Top 0.152: v40.4,11.5 39.6,11.5 39.47,11.63 37.02,11.63 37,11.62 36.5,11.62 36.48,11.63 35.04,11.63 35,11.67 28.65,11.67 28.07,12.25 v27.78,12.25 D185.2 | D11.2 27.76,42.25 v27.78,42.23 | D22.2 27.74,39.25 v27.78,39.21 | D35.2 27.73,36.25 v27.78,36.2 | D171.2 27.71,33.25 v27.78,33.18 | D50.2 v27.77,30.25 v27.78,30.24 | D66.2 27.76,27.25 v27.78,27.23 | D82.2 27.74,24.25 v27.78,24.21 | D98.2 27.72,21.25 v27.78,21.19 | D114.2 v27.77,18.25 v27.78,18.26 | D129.2 v27.77,15.25 v27.78,15.24 | v27.78,3.25 D161.2 | D153.2 27.76,6.25 v27.78,6.27 | D142.2 27.74,9.25 v27.78,9.21 | D3.2 27.78,44.39 v27.78,44.05
  Bottom 0.152: P1.54 43.74,12.49 42.58,11.34 41.55,11.34 41.39,11.5 v40.4,11.5 | v27.78,44.05 v27.78,42.23 v27.78,39.21 v27.78,36.2 v27.78,33.18 v27.78,30.24 v27.78,27.23 v27.78,24.21 v27.78,21.19 v27.78,18.26 v27.78,15.24 v27.78,12.25 v27.78,9.21 v27.78,6.27 v27.78,3.25
C8  (via drill 0.35)
  Top 0.152: D162.2 v24.76,3.25 v24.77,3.25 | v24.84,44.05 24.84,44.33 D4.2 | D12.2 24.74,42.25 v24.77,42.23 | D23.2 24.73,39.25 v24.77,39.21 | D36.2 24.63,36.25 v24.77,36.12 | D172.2 24.69,33.25 v24.77,33.18 | D51.2 24.76,30.25 v24.77,30.24 | D67.2 24.74,27.25 v24.77,27.23 | D83.2 24.64,24.25 v24.77,24.13 25.24,23.65 27.48,23.65 27.53,23.6 28.03,23.6 28.08,23.65 30.42,23.65 30.47,23.6 30.97,23.6 31.02,23.65 33.43,23.65 33.48,23.6 33.99,23.6 34.04,23.65 35.67,23.65 35.68,23.64 36.32,23.64 36.8,24.13 v37.07,24.13 | D99.2 24.71,21.25 v24.77,21.19 | D115.2 v24.77,18.26 | D186.2 24.74,12.25 v24.77,12.22 | D143.2 24.72,9.25 v24.77,9.21 | D154.2 23.95,6.27 v24.77,6.27 | D130.2 24.75,15.25 v24.77,15.24
  Bottom 0.152: P1.53 43.02,10.93 42.41,10.32 40.64,10.32 39.56,9.24 39.56,8.97 39.08,8.49 38.66,8.49 38.34,8.81 38.34,22.86 v37.07,24.13 | v24.77,3.25 v24.77,6.27 v24.77,9.21 v24.77,12.22 v24.77,15.24 v24.77,18.26 v24.77,21.19 v24.77,24.13 v24.77,27.23 v24.77,30.24 v24.77,33.18 v24.77,36.12 v24.77,39.21 v24.77,42.23 24.84,42.31 v24.84,44.05
C9  (via drill 0.35)
  Top 0.152: D163.2 v21.74,3.25 v21.75,3.25 | v21.75,45.01 21.17,45.01 D5.2 | D13.2 21.65,42.25 v21.75,42.15 | D24.2 21.71,39.25 v21.75,39.21 | D37.2 21.69,36.25 v21.75,36.2 | D173.2 v21.74,33.25 v21.75,33.26 | D52.2 v21.74,30.25 v21.75,30.24 | D68.2 21.64,27.25 v21.75,27.15 | D84.2 21.63,24.25 v21.75,24.13 | D100.2 21.61,21.25 v21.75,21.11 | D116.2 21.01,18.34 v21.75,18.34 | D131.2 v21.74,15.25 v21.75,15.24 | D187.2 21.64,12.25 v21.75,12.14 | D144.2 21.71,9.25 v21.75,9.21 22.3,8.66 24.45,8.66 24.51,8.6 25.02,8.6 25.07,8.65 27.48,8.65 27.53,8.6 28.03,8.6 28.07,8.64 33.18,8.64 33.19,8.65 35.67,8.65 35.68,8.64 36.32,8.64 36.72,9.05 v37.15,9.05 | D155.2 20.95,6.27 v21.75,6.27
  Bottom 0.152: P1.52 40.57,9.46 39.25,8.14 | 39.25,8.14 39.21,8.1 | v21.75,3.25 v21.75,6.27 v21.75,9.21 v21.75,12.14 v21.75,15.24 v21.75,18.34 v21.75,21.11 v21.75,24.13 v21.75,27.15 v21.75,30.24 v21.75,33.26 v21.75,36.2 v21.75,39.21 v21.75,42.15 v21.75,45.01 | 39.25,8.14 38.06,8.14 v37.15,9.05
C10  (via drill 0.35)
  Top 0.152: D164.2 18.66,3.25 v18.73,3.17 | v17.94,45.24 D6.2 | D14.2 18.71,42.25 v18.73,42.23 | D25.2 18.69,39.25 v18.73,39.21 | D38.2 18.68,36.25 v18.73,36.2 | D174.2 18.66,33.25 v18.73,33.18 | D53.2 v18.72,30.25 v18.73,30.24 | D69.2 18.63,27.25 v18.73,27.15 | D85.2 18.69,24.25 v18.73,24.21 | D101.2 18.68,21.25 v18.73,21.19 | D117.2 18.66,18.25 v18.73,18.18 19.28,17.63 30.68,17.63 v31.22,18.18 | D132.2 v18.72,15.25 v18.73,15.24 | D188.2 18.71,12.25 v18.73,12.22 | D145.2 18.69,9.25 v18.73,9.21 | D156.2 17.95,6.27 v18.73,6.27
  Bottom 0.152: v18.73,3.17 v18.73,6.27 v18.73,9.21 v18.73,12.22 v18.73,15.24 v18.73,18.18 v18.73,21.19 v18.73,24.21 v18.73,27.15 v18.73,30.24 v18.73,33.18 v18.73,36.2 v18.73,39.21 v18.73,42.23 18.73,43.82 18.24,44.31 18.24,44.94 v17.94,45.24 | P1.51 39.67,8.08 39.29,7.7 38.24,7.7 36.18,5.64 35.25,5.64 34.92,5.32 32.45,5.32 32.15,5.62 32.15,17.25 v31.22,18.18
C11  (via drill 0.35)
  Top 0.152: v30.96,15.16 30.44,14.64 28.04,14.64 28.03,14.63 27.53,14.63 27.52,14.64 25.03,14.64 25.02,14.63 24.51,14.63 24.5,14.64 22.01,14.64 22,14.63 21.5,14.63 21.49,14.64 18.99,14.64 18.98,14.63 18.48,14.63 18.47,14.64 16.68,14.64 16.08,15.25 v15.8,15.25 | D157.2 15.74,6.25 v15.8,6.19 | v15.8,42.23 15.77,42.25 D15.2 | D26.2 15.76,39.25 v15.8,39.21 | D39.2 15.74,36.25 v15.8,36.2 | D175.2 15.79,33.25 v15.8,33.26 | D54.2 15.71,30.25 v15.8,30.16 | D70.2 15.77,27.25 v15.8,27.23 | D86.2 14.96,24.29 v15.8,24.29 | D102.2 15.74,21.25 v15.8,21.19 | D118.2 v15.8,18.26 | D189.2 15.77,12.25 v15.8,12.22 | D133.2 v15.8,15.25 | v15.8,15.25 v15.8,15.24 | D146.2 14.96,9.29 v15.8,9.29
  Bottom 0.152: v30.96,15.16 31.83,14.29 31.83,5.51 32.35,4.99 35.23,4.99 35.58,5.34 36.31,5.34 37.77,6.8 P1.50 | v15.8,6.19 v15.8,9.29 v15.8,12.22 v15.8,15.24 v15.8,18.26 v15.8,21.19 v15.8,24.29 v15.8,27.23 v15.8,30.16 v15.8,33.26 v15.8,36.2 v15.8,39.21 v15.8,42.23
C12  (via drill 0.35)
  Top 0.152: v12.78,42.23 11.95,42.23 D16.2 | D27.2 12.74,39.25 v12.78,39.21 | D40.2 11.95,36.27 v12.78,36.27 | D176.2 v12.77,33.25 v12.78,33.26 | D55.2 12.69,30.25 v12.78,30.16 | D71.2 12.68,27.25 v12.78,27.15 | D87.2 11.96,24.29 v12.78,24.29 | D103.2 12.72,21.25 v12.78,21.19 | D119.2 12.71,18.25 v12.78,18.18 | D134.2 12.69,15.25 v12.78,15.16 | D190.2 12.67,12.25 v12.78,12.14 | D147.2 v11.99,9.25 | P1.48 34.98,4.6 33.48,3.1 33.48,2.81 33.27,2.59 30.8,2.59 29.95,1.74 19.31,1.74 18.38,2.67 16.66,2.67 13.96,5.37 12.81,5.37 D158.2 v12.01,6.33
  Bottom 0.152: v12.78,42.23 v12.78,39.21 v12.78,36.27 v12.78,33.26 v12.78,30.16 v12.78,27.15 v12.78,24.29 v12.78,21.19 v12.78,18.18 v12.78,15.16 v12.78,12.14 11.99,11.35 v11.99,9.25 12.01,9.23 v12.01,6.33
  other vias: 37.42,4.6
C13  (via drill 0.35)
  Top 0.152: D148.2 9.81,9.25 | 9.81,9.25 v9.84,9.29 | v9.76,39.29 9.72,39.25 D28.2 | D191.2 9.66,12.25 v9.76,12.14 | D135.2 v9.75,15.25 v9.76,15.24 | D120.2 9.69,18.25 v9.76,18.18 | D104.2 9.71,21.25 v9.76,21.19 | D88.2 9.72,24.25 v9.76,24.21 | D72.2 9.74,27.25 v9.76,27.23 | D56.2 9.68,30.25 v9.76,30.16 | D177.2 v9.76,33.25 v9.76,33.26 | D41.2 9.71,36.25 v9.76,36.2 | v31.11,6.19 30.56,5.63 24.45,5.63 24.45,5.64 16.1,5.64 16.05,5.58 15.54,5.58 15.46,5.67 13.52,5.67 v12.92,6.27 | v12.94,9.21 12.88,9.21 12.32,8.64 10.41,8.64 9.81,9.25
  Bottom 0.152: v9.84,9.29 9.84,10 9.76,10.08 v9.76,12.14 v9.76,15.24 v9.76,18.18 v9.76,21.19 v9.76,24.21 v9.76,27.23 v9.76,30.16 v9.76,33.26 v9.76,36.2 v9.76,39.29 | P1.49 37.04,5.64 36.08,4.68 32.23,4.68 31.11,5.79 v31.11,6.19 | v12.92,6.27 12.92,9.19 v12.94,9.21
C14  (via drill 0.35)
  Top 0.152: D42.2 5.95,36.27 v6.75,36.27 | D192.2 5.95,12.22 v6.75,12.22 6.75,9.53 11.27,5 13.89,5 16.63,2.26 18.36,2.26 19.18,1.43 30.08,1.43 30.88,2.23 33.34,2.23 33.78,2.68 33.78,2.94 34.51,3.66 35.76,3.66 P1.47 | D136.2 6.74,15.25 v6.75,15.24 | D121.2 v6.75,18.26 | D105.2 6.69,21.25 v6.75,21.19 | D89.2 6.71,24.25 v6.75,24.21 | D73.2 6.64,27.25 v6.75,27.15 | D57.2 v6.74,30.25 v6.75,30.24 | D178.2 6.68,33.25 v6.75,33.18
  Bottom 0.152: v6.75,36.27 v6.75,33.18 v6.75,30.24 v6.75,27.15 v6.75,24.21 v6.75,21.19 v6.75,18.26 v6.75,15.24 v6.75,12.22
  other vias: 35.78,3.69
C15  (via drill 0.35)
  Top 0.152: D58.2 2.92,29.83 2.62,29.53 1.75,29.53 1.46,29.24 1.46,28.5 1.52,28.44 1.52,26.51 | 1.52,20.63 1.52,17.8 1.96,17.36 2.86,17.36 | D74.2 2.92,26.74 2.7,26.51 1.52,26.51 | D90.2 2.92,23.72 2.7,23.5 1.52,23.5 | D106.2 2.92,20.94 2.62,20.63 1.52,20.63 | 2.86,17.36 3.75,17.36 4.45,16.67 4.45,11.4 11.14,4.7 13.77,4.7 16.51,1.96 18.23,1.96 19.06,1.13 30.22,1.13 31.02,1.93 33.47,1.93 33.82,2.29 33.83,2.29 34.29,2.74 v34.55,2.74 | D122.2 2.92,17.43 2.86,17.36 | 1.52,20.63 1.52,23.5 | 1.52,23.5 1.52,26.51
  Bottom 0.152: P1.46 34.23,2.74 v34.55,2.74
G0  (via drill 0.35)
  Top 0.152: D1.4 31.5,46.17 29.21,46.17 | 29.21,46.17 29.05,46.17 29.07,46.2 D2.4 | D4.4 23.07,46.2 23.1,46.17 | 26.11,46.17 26.07,46.21 D3.4 v26.07,46.67 | 23.1,46.17 23.65,46.17 23.69,46.13 24.47,46.13 24.48,46.13 25.21,46.13 25.25,46.17 26.11,46.17 | 29.21,46.17 29.18,46.2 28.81,46.2 28.77,46.16 27.4,46.16 27.39,46.17 26.11,46.17 | D6.4 17.05,46.73 17.05,46.23 17.33,45.95 18.33,45.95 18.43,45.84 19.19,45.84 19.52,46.17 20,46.17 | 23.1,46.17 20,46.17 | D5.4 20.07,46.24 20,46.17
  Bottom 0.152: P1.1 25,47.74 25.09,47.65 25.45,47.3 v26.07,46.67
G1  (via drill 0.35)
  Top 0.152: D16.4 11.07,43.6 11.51,43.17 14.05,43.17 | D7.4 37.5,43.17 35.08,43.17 | 14.05,43.17 16.99,43.17 | 20.08,43.17 23.18,43.17 | 29.13,43.17 31.99,43.17 | 31.99,43.17 35.08,43.17 | D8.4 35.08,43.17 | D9.4 32.08,43.26 31.99,43.17 | D10.4 29.07,43.23 29.13,43.17 | D11.4 26.07,43.21 26.11,43.17 | D12.4 23.07,43.27 23.18,43.17 | D13.4 | D13.4 20.07,43.18 20.08,43.17 | D14.4 17.07,43.26 16.99,43.17 | D15.4 14.07,43.2 14.05,43.17 | D13.4 | 16.99,43.17 17.65,43.17 17.68,43.14 18.18,43.14 18.21,43.17 20.08,43.17 | 23.18,43.17 24.44,43.17 24.47,43.14 25.22,43.14 25.25,43.17 26.11,43.17 | 26.11,43.17 27.37,43.17 27.4,43.14 28.62,43.14 28.65,43.17 29.13,43.17
  Bottom 0.152: P1.4 19.41,48.27 18.18,47.04 18.18,46.51 19.16,45.53 19.16,44.66 D13.4
  other vias: 20.07,43.75
G2  (via drill 0.35)
  Top 0.152: D28.4 8.07,40.9 8.51,41.33 11.11,41.33 | D17.4 40.5,41.33 38.02,41.33 | 14.13,41.33 17.07,41.33 | 17.07,41.33 20.08,41.33 | 20.08,41.33 23.1,41.33 | 23.1,41.33 26.11,41.33 | 26.11,41.33 29.13,41.33 | 29.13,41.33 32.07,41.33 | 32.07,41.33 35.08,41.33 | 35.08,41.33 38.02,41.33 | D18.4 38.02,40.8 38.02,41.33 | D19.4 35.08,41.32 35.08,41.33 | D20.4 32.08,41.32 32.07,41.33 | D21.4 29.07,41.27 29.13,41.33 | D22.4 26.07,41.29 26.11,41.33 | D23.4 23.07,41.3 23.1,41.33 | D24.4 20.07,41.32 20.08,41.33 | D25.4 17.07,41.32 17.07,41.33 | D26.4 | 14.13,41.33 14.07,41.27 D26.4 | D27.4 11.07,41.29 11.11,41.33 | D26.4 | 11.11,41.33 11.65,41.33 11.68,41.36 12.18,41.36 12.21,41.33 14.13,41.33
  Bottom 0.152: P1.7 14.12,40.8 D26.4
  other vias: 14.07,40.75
G3  (via drill 0.35)
  Top 0.152: D42.4 5.08,37.6 5.5,37.17 6.36,37.17 6.37,37.19 7.12,37.19 7.14,37.17 8.02,37.17 | D29.4 43.5,37.17 41.04,37.17 | 14.21,37.17 16.99,37.17 | 16.99,37.17 20,37.17 | 20,37.17 23.1,37.17 | 23.1,37.17 26.04,37.17 | 26.04,37.17 29.13,37.17 | 29.13,37.17 32.15,37.17 | 32.15,37.17 35,37.17 | 35,37.17 38.1,37.17 | 38.1,37.17 41.04,37.17 | D30.4 41.08,37.21 41.04,37.17 | D31.4 38.08,37.2 38.1,37.17 | D32.4 35.08,37.24 35,37.17 | D33.4 32.08,37.24 32.15,37.17 | D34.4 29.07,37.23 29.13,37.17 | D35.4 26.07,37.21 26.04,37.17 | D36.4 23.07,37.2 23.1,37.17 | D37.4 20.07,37.24 20,37.17 | D38.4 17.07,37.26 16.99,37.17 | D39.4 14.07,37.3 14.21,37.17 | D40.4 v11.07,37.7 | v11.07,37.7 11.07,37.21 11.03,37.17 | D41.4 8.07,37.23 8.02,37.17 | 11.03,37.17 12.39,37.17 12.4,37.19 13.16,37.19 13.17,37.17 14.21,37.17 | v11.07,37.7 | 8.02,37.17 8.65,37.17 8.68,37.14 9.18,37.14 9.21,37.17 11.03,37.17
  Bottom 0.152: P1.10 10.4,42.33 10.4,38.37 v11.07,37.7
G4  (via drill 0.35)
  Top 0.152: D178.4 5.08,34.6 5.51,34.16 6.2,34.16 6.21,34.17 8.1,34.17 | D165.4 43.5,34.17 41.12,34.17 | 8.1,34.17 11.11,34.17 | 11.11,34.17 14.05,34.17 | 14.05,34.17 17.14,34.17 | 17.14,34.17 20.08,34.17 | 20.08,34.17 23.1,34.17 | 23.1,34.17 26.11,34.17 | 26.11,34.17 29.13,34.17 | 29.13,34.17 32.07,34.17 | 32.07,34.17 35.08,34.17 | 35.08,34.17 38.1,34.17 | 38.1,34.17 41.12,34.17 | D166.4 41.12,34.71 41.12,34.17 | D167.4 38.1,34.73 38.1,34.17 | D168.4 35.08,34.18 35.08,34.17 | D169.4 32.08,34.18 32.07,34.17 | D170.4 29.07,34.23 29.13,34.17 | D171.4 26.11,34.71 26.11,34.17 | D172.4 23.1,34.73 23.1,34.17 | D173.4 20.07,34.18 20.08,34.17 | D174.4 17.07,34.24 17.14,34.17 | D175.4 14.07,34.2 14.05,34.17 | D176.4 11.11,34.71 11.11,34.17 | D177.4 8.1,34.73 8.1,34.66 | v8.07,34.69 8.1,34.66 | 8.1,34.66 8.1,34.17
  Bottom 0.152: P1.13 7.46,37.31 7.46,35.29 v8.07,34.69
G5  (via drill 0.35)
  Top 0.152: D43.4 46.5,31.17 44.13,31.17 | D58.4 2.08,31.6 2.5,31.17 2.65,31.17 2.68,31.14 3.18,31.14 3.21,31.17 3.97,31.17 | 44.13,31.17 41.04,31.17 | 41.04,31.17 37.94,31.17 | 37.94,31.17 35.08,31.17 | 35.08,31.17 32.07,31.17 | 32.07,31.17 29.05,31.17 | 29.05,31.17 26.04,31.17 | 26.04,31.17 23.1,31.17 | 23.1,31.17 20.08,31.17 | 20.08,31.17 17.07,31.17 | 17.07,31.17 14.13,31.17 | 14.13,31.17 11.11,31.17 | 11.11,31.17 8.1,31.17 | 8.1,31.17 5.08,31.17 | D55.4 11.11,31.71 11.11,31.17 | D54.4 14.13,31.7 14.13,31.17 | D53.4 17.07,31.18 17.07,31.17 | D52.4 20.08,31.74 20.08,31.17 | D51.4 23.1,31.73 23.1,31.17 | D50.4 26.07,31.21 26.04,31.17 | D48.4 32.08,31.18 32.07,31.17 | D47.4 35.08,31.17 | D46.4 38.08,31.3 37.94,31.17 | D44.4 44.08,31.23 44.13,31.17 | D49.4 29.07,31.97 29.13,32.02 29.13,31.25 29.05,31.17 | D45.4 41.08,31.21 41.04,31.17 | 5.08,31.17 D57.4 | D56.4 8.1,31.73 8.1,31.17 | 5.08,31.17 3.97,31.17 | v3.97,31.67 3.97,31.17
  Bottom 0.152: P1.16 3.97,33.13 v3.97,31.67
G6  (via drill 0.35)
  Top 0.152: D59.4 46.5,28.17 44.05,28.17 | 5.08,28.17 8.1,28.17 | 8.1,28.17 11.03,28.17 | 11.03,28.17 14.13,28.17 | 14.13,28.17 17.07,28.17 | 17.07,28.17 20.16,28.17 | 20.16,28.17 23.1,28.17 | 23.1,28.17 26.11,28.17 | 26.11,28.17 29.05,28.17 | 29.05,28.17 32.07,28.17 | 32.07,28.17 35,28.17 | 35,28.17 38.02,28.17 | 38.02,28.17 41.04,28.17 | 41.04,28.17 44.05,28.17 | D73.4 5.08,28.17 | D72.4 8.1,28.73 8.1,28.17 | D71.4 11.07,28.21 11.03,28.17 | D70.4 14.13,28.7 14.13,28.17 | D69.4 17.07,28.18 17.07,28.17 | D68.4 20.16,28.66 20.16,28.17 | D67.4 23.1,28.73 23.1,28.17 | D60.4 44.08,28.19 44.05,28.17 | D61.4 41.08,28.21 41.04,28.17 | D62.4 38.08,28.23 38.02,28.17 | D63.4 35.08,28.24 35,28.17 | D64.4 32.08,28.18 32.07,28.17 | D65.4 29.07,28.2 29.05,28.17 | D66.4 26.11,28.71 26.11,28.17 | v2.07,28.75 D74.4 2.08,28.6 2.53,28.14 3.23,28.14 3.26,28.17 5.08,28.17
  Bottom 0.152: v2.07,28.75 1.4,28.75 P1.19
G7  (via drill 0.35)
  Top 0.152: D75.4 46.5,25.17 44.13,25.17 | D90.4 2.08,25.6 2.5,25.17 3.89,25.17 | 44.13,25.17 41.2,25.17 | 41.2,25.17 38.02,25.17 | 38.02,25.17 35.16,25.17 | 35.16,25.17 32.23,25.17 | 32.23,25.17 29.13,25.17 | 29.13,25.17 26.04,25.17 | 26.04,25.17 23.02,25.17 | 23.02,25.17 20,25.17 | 20,25.17 17.14,25.17 | 11.11,25.17 8.18,25.17 | 8.18,25.17 5.08,25.17 | 5.08,25.17 3.89,25.17 | D89.4 5.08,25.17 | D86.4 14.07,25.2 14.05,25.17 | D87.4 11.11,25.71 11.11,25.17 | D88.4 8.18,25.65 8.18,25.17 | D85.4 17.07,25.24 17.14,25.17 | D84.4 20.07,25.24 20,25.17 | D76.4 44.13,25.69 44.13,25.17 | D77.4 41.2,25.63 41.2,25.17 | D78.4 38.08,25.23 38.02,25.17 | D79.4 35.16,25.66 35.16,25.17 | D80.4 32.23,25.6 32.23,25.17 | D81.4 29.13,25.69 29.13,25.17 | D82.4 26.07,25.21 26.04,25.17 | D83.4 23.07,25.23 23.02,25.17 | 17.14,25.17 16.2,25.17 16.17,25.2 15.42,25.2 15.39,25.17 14.05,25.17 | 14.05,25.17 13.19,25.17 13.16,25.2 12.4,25.2 12.37,25.17 11.11,25.17 | v3.89,25.72 3.89,25.17
  Bottom 0.152: P1.22 3.57,25.72 v3.89,25.72
G8  (via drill 0.35)
  Top 0.152: D106.4 2.08,22.6 2.5,22.17 3.81,22.17 | 41.04,22.17 38.1,22.17 | 32.15,22.17 29.13,22.17 | 29.13,22.17 26.11,22.17 | 26.11,22.17 23.02,22.17 | 23.02,22.17 20,22.17 | 20,22.17 17.14,22.17 | 17.14,22.17 14.05,22.17 | 14.05,22.17 11.11,22.17 | 11.11,22.17 8.1,22.17 | 5.08,22.17 3.81,22.17 | D105.4 5.08,22.17 | D104.4 8.1,22.73 8.1,22.17 | D103.4 11.11,22.71 11.11,22.17 | D102.4 14.07,22.2 14.05,22.17 | D101.4 17.14,22.68 17.14,22.17 | D100.4 20.07,22.24 20,22.17 | D99.4 23.07,22.23 23.02,22.17 | D98.4 26.07,22.21 26.11,22.17 | D96.4 32.15,22.68 32.15,22.17 | D97.4 29.13,22.69 29.13,22.17 | D95.4 35.08,22.24 35,22.17 | D94.4 38.1,22.73 38.1,22.17 | D93.4 41.08,22.21 41.04,22.17 | 44.13,22.69 D92.4 44.08,22.19 44.05,22.17 | 41.04,22.17 44.05,22.17 | D91.4 45.92,22.75 45.34,22.17 44.05,22.17 | 38.1,22.17 37.14,22.17 37.13,22.18 36.37,22.18 36.36,22.17 35,22.17 | 35,22.17 34.53,22.17 34.52,22.18 33.76,22.18 33.75,22.17 32.15,22.17 | v3.78,22.7 3.81,22.67 3.81,22.17 | 8.1,22.17 6.21,22.17 6.18,22.14 5.68,22.14 5.65,22.17 5.08,22.17
  Bottom 0.152: P1.25 3.17,18.71 3.17,22.1 v3.78,22.7
G9  (via drill 0.35)
  Top 0.152: D122.4 2.08,19.9 2.5,20.33 5.08,20.33 | 8.02,20.33 11.11,20.33 | 11.11,20.33 14.13,20.33 | 14.13,20.33 16.99,20.33 | 16.99,20.33 20.08,20.33 | 20.08,20.33 23.1,20.33 | 23.1,20.33 26.19,20.33 | 26.19,20.33 29.13,20.33 | 29.13,20.33 32.15,20.33 | 32.15,20.33 35,20.33 | 44.13,20.33 41.51,20.33 41.08,19.9 D109.4 40.96,19.63 39.9,19.63 39.61,19.92 39.61,20.06 39.34,20.33 38.1,20.33 | D108.4 44.13,19.81 44.13,20.33 | D110.4 38.08,20.3 38.1,20.33 | D111.4 35.08,20.26 35,20.33 | D112.4 32.08,20.26 32.15,20.33 | D113.4 29.07,20.27 29.13,20.33 | D114.4 26.07,20.21 26.19,20.33 | D115.4 23.07,20.3 23.1,20.33 | D116.4 20.07,20.32 20.08,20.33 | D117.4 17.07,20.24 16.99,20.33 | D118.4 14.07,20.27 14.13,20.33 | D119.4 11.07,20.29 11.11,20.33 | D120.4 8.07,20.27 8.02,20.33 | D121.4 5.08,19.8 | 5.08,20.33 5.08,20.32 5.08,19.8 | 44.13,20.33 45.34,20.33 45.51,20.16 45.51,19.91 45.87,19.55 46.88,19.55 D107.4 | 5.08,20.33 5.65,20.33 5.68,20.36 6.18,20.36 6.21,20.33 8.02,20.33 | v5.02,19.75 5.08,19.8 | 35,20.33 38.1,20.33
  Bottom 0.152: P1.28 5.02,13.09 v5.02,19.75
G10  (via drill 0.35)
  Top 0.152: D136.4 5.08,16.9 5.5,17.33 8.1,17.33 | 10.95,17.33 14.05,17.33 | 14.05,17.33 17.07,17.33 | 17.07,17.33 20,17.33 | 20,17.33 23.02,17.33 | 23.02,17.33 26.11,17.33 | 26.11,17.33 29.13,17.33 | 32.07,17.33 35,17.33 | 35,17.33 38.18,17.33 | 38.18,17.33 41.04,17.33 | 8.1,17.33 8.07,17.31 D135.4 8.07,16.77 v8.02,16.83 | D134.4 10.95,16.87 10.95,17.33 | D133.4 14.13,16.7 14.13,16.48 14.05,16.56 14.05,17.33 | D132.4 17.07,17.33 | D131.4 20.07,17.26 20,17.33 | D130.4 23.02,16.81 23.02,17.33 | D129.4 26.07,17.29 26.11,17.33 | D128.4 29.07,17.27 29.13,17.33 | D127.4 32.07,16.76 32.07,17.33 | D126.4 35,16.82 35,17.33 | D125.4 38.08,17.22 38.18,17.33 | D124.4 41.04,16.79 41.04,17.33 | D123.4 43.93,16.89 43.15,16.89 42.85,17.2 42.48,17.2 42.34,17.33 41.04,17.33 | 8.1,17.33 8.65,17.33 8.68,17.36 9.18,17.36 9.21,17.33 10.95,17.33 | 29.13,17.33 32.07,17.33
  Bottom 0.152: P1.31 7.98,16.79 v8.02,16.83
G11  (via drill 0.35)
